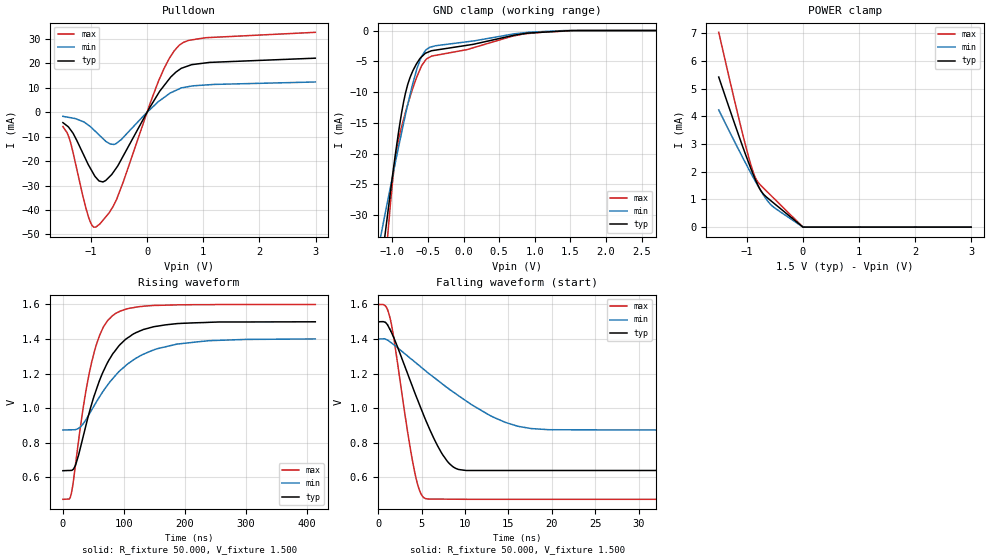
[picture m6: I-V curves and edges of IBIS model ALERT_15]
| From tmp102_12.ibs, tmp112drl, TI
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|   ALERT_15   1.8V digital open-drain Model
[Model] ALERT_15
Model_type   Open_drain
| Signals   ALERT(3)
Polarity   Non-Inverting
Enable   Active-Low
Vmeas = 0.75
Vref = 0.75
Cref = 15pF
Rref = 50
|   typ   min   max
|   (nom PVT)   (Fast PVT)   (slow PVT)
|   output low
|C_comp   1.1288980e-10   7.0765000e-11   1.4519290e-10
| Where   nom PVT is  Nominal Process, 1.5V, -40C
|   Fast PVT is Strong Process, 1.6V, 125C
|   Slow PVT is Weak Process, 1.4V, 27C
|   output high
C_comp   1.2879940e-12  1.2276710e-12  1.3887450e-12
| Where   nom PVT is  Nominal Process, 1.5V, 27C
|   Fast PVT is Strong Process, 1.6V, -40C
|   Slow PVT is Weak Process, 1.4V, 125C
[Voltage Range]   1.5   1.4   1.6
[Temperature Range]   27   125   -40
|Ambient Temperature   27   125   -40
[Pullup Reference]   1.5   1.4   1.6
[Pulldown Reference]   0   0   0
[Power Clamp Reference]   1.5   1.4   1.6
[GND Clamp Reference]   0   0   0
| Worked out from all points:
|   slope of the pulldown table from 0 to 0.225 V, typ, clamps not added: 26.2 ohm
|   POWER clamp passes 1 mA (typ) near -0.60 V on its own axis
|   falling waveform, R_fixture 50.000, V_fixture 1.500: 20-80 % time 4.12ns typ, 8.61ns min, 2.05ns max; typ from 1.5 V to 0.639 V
|   rising waveform, R_fixture 50.000, V_fixture 1.500: 20-80 % time 53.2ns typ, 77.5ns min, 34ns max; typ from 0.639 V to 1.5 V
[Pulldown]
|   Voltage   I(typ)   I(min)   I(max)
-1.5V     -4.294mA   -1.72mA    -5.901mA
-1.364V   -7.208mA   -2.279mA   -12.34mA
-1.044V   -21.64mA   -5.369mA   -42.9mA
-979.5mV  -24.23mA   -6.594mA   -46.37mA
-916.7mV  -26.59mA   -7.97mA    -47.03mA
-785.6mV  -28.53mA   -10.85mA   -44.18mA
-559.2mV  -23.18mA   -12.97mA   -36.4mA
195.8mV   7.482mA    4.197mA    12.3mA
392mV     13.5mA     7.505mA    21.84mA
570mV     17.3mA     9.501mA    27.3mA
1.04V     20.12mA    11.1mA     30.43mA
2.995V    22.06mA    12.33mA    32.63mA
[GND Clamp]
|   Voltage   I(typ)   I(min)   I(max)
-1.5V     -72.01mA   -53.62mA   -104.5mA
-1.156V   -38.18mA   -32.94mA   -46.94mA
-1.109V   -33.61mA   -30.1mA    -39.54mA
-1.064V   -29.48mA   -27.45mA   -32.92mA
-990.4mV  -22.83mA   -23.25mA   -23.72mA
-941.6mV  -18.71mA   -20.45mA   -19.45mA
-845.9mV  -11.76mA   -15.21mA   -14.52mA
-787.5mV  -8.856mA   -12.16mA   -12.12mA
-594.6mV  -4.317mA   -4.285mA   -5.832mA
-473.2mV  -3.387mA   -2.714mA   -4.304mA
859.2mV   -492.7uA   -350.6uA   -531.4uA
2.995V    0A         0A         0A
[POWER Clamp]
|   Voltage   I(typ)   I(min)   I(max)
-1.5V     5.425mA    4.236mA    7.042mA
-1.244V   3.9mA      3.195mA    4.799mA
-1.064V   2.856mA    2.475mA    3.282mA
-937.8mV  2.169mA    1.99mA     2.325mA
-852.3mV  1.74mA     1.672mA    1.81mA
-809.3mV  1.545mA    1.518mA    1.647mA
-736.9mV  1.278mA    1.269mA    1.48mA
-652.4mV  1.09mA     1.006mA    1.309mA
-579.5mV  965.9uA    825.9uA    1.163mA
-415.8mV  692.8uA    567.6uA    834.4uA
1.403mV   -2.342uA   -1.912uA   -2.819uA
2.995V    -2.342uA   -1.912uA   -2.819uA
[Ramp]
R_load = 50
|   typ   min   max
dV/dt_r   0.509358/5.29209e-008   0.30642/7.7264e-008   0.675795/3.38992e-008
dV/dt_f   0.509358/4.12051e-009   0.30642/8.5654e-009   0.675795/2.04387e-009
[Falling Waveform]
R_fixture = 50.000
V_fixture = 1.500
V_fixture_min = 1.400
V_fixture_max = 1.600
C_fixture = 0.000
|  time   V(typ)   V(min)   V(max)
0s        1.5V       1.401V     1.6V
1.348ns   1.457V     1.385V     1.526V
4.231ns   1.088V     1.267V     624.8mV
4.934ns   998.5mV    1.238V     504.6mV
5.742ns   900.2mV    1.205V     475.5mV
7.427ns   731.5mV    1.139V     474.9mV
9.272ns   646.2mV    1.072V     474.2mV
14.61ns   640.5mV    919.2mV    473.7mV
19.83ns   640.4mV    876.1mV    473.7mV
413.8ns   639.2mV    874.7mV    473.7mV
[Rising Waveform]
R_fixture = 50.000
V_fixture = 1.500
V_fixture_min = 1.400
V_fixture_max = 1.600
C_fixture = 0.000
|  time   V(typ)   V(min)   V(max)
0s        639.2mV    874.7mV    473.7mV
13.89ns   640.9mV    875.6mV    508mV
21.07ns   675mV      877.4mV    685.5mV
35ns      861.5mV    919.6mV    1.042V
51.65ns   1.076V     1.017V     1.329V
66.26ns   1.214V     1.1V       1.469V
81.4ns    1.313V     1.17V      1.536V
120.6ns   1.439V     1.291V     1.585V
188.2ns   1.49V      1.372V     1.598V
413.8ns   1.5V       1.401V     1.6V
